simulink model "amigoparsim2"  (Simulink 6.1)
settings: Solver=ode23s  StartTime=0.0  StopTime=400  MaxStep=0.05  RelTol=1e-8
undefined symbols (not defined in the file or in its folder): sys_tf, totaldelay
libraries: simulink x1, cstblocks x1

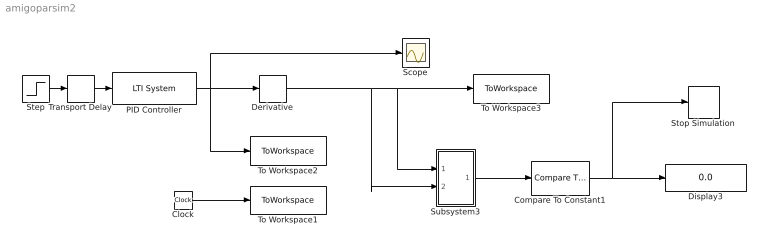
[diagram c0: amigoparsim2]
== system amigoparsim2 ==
  Clock : Clock
  Compare To Constant1 : simulink/Logic and Bit Operations/Compare To Constant  relop=<=  const=0.000001  LogicOutDataTypeMode=boolean  ZeroCross=off
  Derivative : Derivative
  Display3 : Display
  PID Controller : cstblocks/LTI System  sys=syst  IC=[]
  Scope : Scope
  Step : Step  Time=0  SampleTime=0
  Stop Simulation : Stop
  Subsystem3 : Subsystem
  To Workspace1 : ToWorkspace  VariableName=tid  SampleTime=-1  SaveFormat=Array
  To Workspace2 : ToWorkspace  VariableName=step_vals  SampleTime=-1  SaveFormat=Array
  To Workspace3 : ToWorkspace  VariableName=imp_vals  SampleTime=-1  SaveFormat=Array
  Transport Delay : TransportDelay  DelayTime=totaldelay(sys_tf)  BufferSize=100000
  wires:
  Clock/1 -> To Workspace1/1
  Step/1 -> Transport Delay/1
  PID Controller/1 -> To Workspace2/1, Derivative/1, Scope/1
  Derivative/1 -> To Workspace3/1, Subsystem3/1(In1), Subsystem3/2(In2)
  Subsystem3/1(Out1) -> Compare To Constant1/1
  Compare To Constant1/1 -> Display3/1, Stop Simulation/1
  Transport Delay/1 -> PID Controller/1

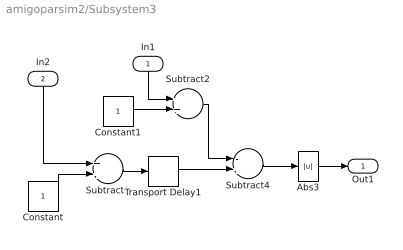
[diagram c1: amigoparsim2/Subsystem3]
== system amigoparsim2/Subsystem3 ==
  In1 : Inport  Orientation=down  Port=1  LatchInput=off
  In2 : Inport  Orientation=down  Port=2  LatchInput=off
  Abs3 : Abs  ZeroCross=off
  Constant : Constant
  Constant1 : Constant
  Subtract1 : Sum  OutScaling=2^-10
  Subtract2 : Sum  OutScaling=2^-10
  Subtract4 : Sum  Inputs=-+  OutScaling=2^-10
  Transport Delay1 : TransportDelay  DelayTime=50  BufferSize=10000
  Out1 : Outport
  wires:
  Abs3/1 -> Out1/1
  Subtract4/1 -> Abs3/1
  Transport Delay1/1 -> Subtract4/2
  Constant/1 -> Subtract1/2
  In2/1 -> Subtract1/1
  Subtract1/1 -> Transport Delay1/1
  Constant1/1 -> Subtract2/2
  Subtract2/1 -> Subtract4/1
  In1/1 -> Subtract2/1
